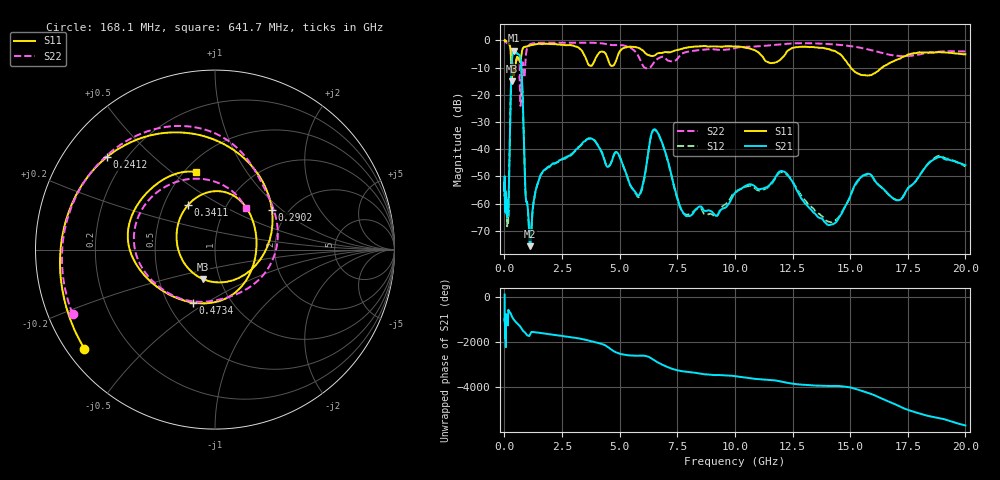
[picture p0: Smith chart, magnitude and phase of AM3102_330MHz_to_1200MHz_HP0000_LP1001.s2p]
! Date/Time: Tue, Sep 11, 2018 5:08 PM
! Network Analyzer: Agilent Technologies E8362B Rev: A.07.50.63
! Sweep from 0.010 to 20.000 GHz, 1601 Points, Sweep Type: LOG
! Power Supply: 4.950 V, 0.001 A
# Hz S DB R 50
!freq MagS11 AngS11 MagS21 AngS21 MagS12 AngS12 MagS22 AngS22
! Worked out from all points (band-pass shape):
!   1601 points, 10 MHz to 20 GHz, reference 50 ohm
!   highest |S21| = -3.70 dB at 432.6 MHz (marker M1); lowest = -75.7 dB at 1.108 GHz (marker M2)
!   |S21| within 3 dB of the highest: 328 MHz to 701.5 MHz (373.5 MHz wide, 72.6 % of centre)
!   lowest |S11| = -15.0 dB at 314.7 MHz (marker M3), VSWR 1.43, Z = 41.5 - j14.1 ohm
!   |S11| at or under -10 dB: 295.3 MHz to 349.1 MHz (53.7 MHz wide, 16.7 % of centre); 368.5 MHz to 471.8 MHz (103.3 MHz wide, 24.6 % of centre); 15.03 GHz to 16.38 GHz (1.353 GHz wide, 8.62 % of centre)
!   |S22| runs from -24.1 to -0.3 dB; largest |S21 - S12| = 0.012
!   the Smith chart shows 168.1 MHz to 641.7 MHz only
!   S11 on the Smith chart (normalised r, x): 168.1 MHz: 0.05, -0.34; 241.2 MHz: 0.13, +0.36; 290.2 MHz: 1.65, +0.86; 341.1 MHz: 0.66, +0.36; 473.4 MHz: 0.67, -0.44; 641.7 MHz: 0.57, +0.61
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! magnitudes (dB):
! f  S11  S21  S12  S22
! 10 MHz  0.0  -53.8  -52.4  -0.3
! 35.55 MHz  0.0  -58.9  -60.8  -0.5
! 126.4 MHz  -0.4  -62.3  -65.9  -1.0
! 168.1 MHz  -0.8  -64.2  -65.6  -1.2
! 241.2 MHz  -2.0  -34.7  -34.8  -1.8
! 290.2 MHz  -8.2  -14.2  -14.3  -3.6
! 314.7 MHz  -15.0  -8.2  -8.2  -6.0
! 341.1 MHz  -10.7  -5.8  -5.9  -8.1
! 432.6 MHz  -12.1  -3.7  -3.8  -10.5
! 447.2 MHz  -11.2  -3.7  -3.8  -9.9
! 473.4 MHz  -9.9  -3.8  -3.9  -8.8
! 641.7 MHz  -7.0  -5.2  -5.3  -10.9
! 702.3 MHz  -7.5  -6.7  -6.8  -24.1
! 1.108 GHz  -1.8  -75.7  -74.9  -1.4
! 1.59 GHz  -1.3  -49.1  -49.4  -0.8
! 3.757 GHz  -9.3  -36.0  -36.0  -0.8
! 5.652 GHz  -2.4  -55.4  -55.7  -3.9
! 6.549 GHz  -5.4  -32.8  -33.0  -7.4
! 7.958 GHz  -2.5  -64.6  -64.0  -4.1
! 12.03 GHz  -6.5  -48.0  -48.4  -1.4
! 14.14 GHz  -3.4  -67.8  -66.8  -1.3
! 20 GHz  -5.1  -45.9  -46.3  -4.0
